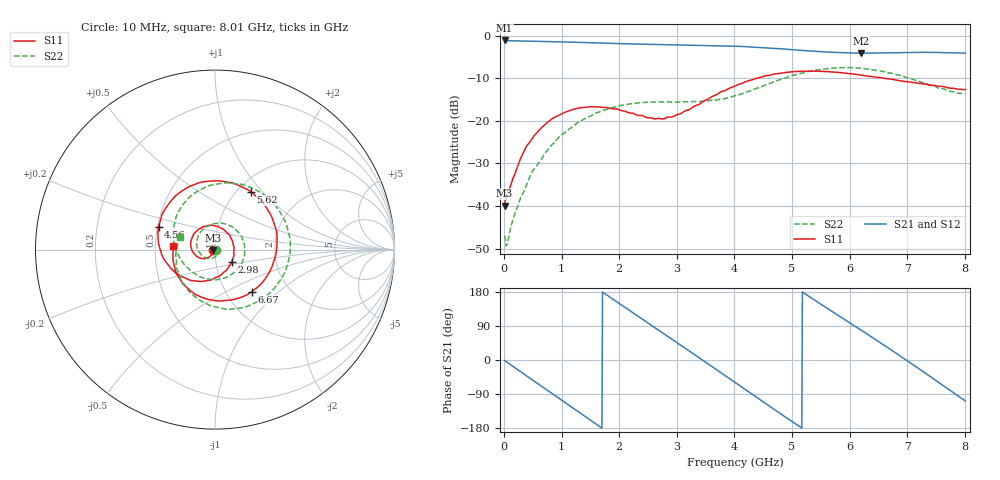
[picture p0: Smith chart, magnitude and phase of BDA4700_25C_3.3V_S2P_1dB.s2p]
!Agilent Technologies,E5071B,MY42404982,A.09.10
!Date: Mon Oct 20 18:03:23 2025
!Data & Calibration Information:
!Freq	S11:SOLT2(ON)	S21:SOLT2(ON)	S12:SOLT2(ON)	S22:SOLT2(ON)
# Hz S RI R 50
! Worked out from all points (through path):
!   801 points, 10 MHz to 8.01 GHz, reference 50 ohm
!   highest |S21| = -1.12 dB at 10 MHz (marker M1); lowest = -4.1 dB at 6.2 GHz (marker M2)
!   group delay of S21, straight-line fit = 286 ps
!   lowest |S11| = -39.9 dB at 10 MHz (marker M3), VSWR 1.02, Z = 49 - j0.224 ohm
!   |S11| at or under -10 dB: start of sweep to 4.387 GHz; 6.606 GHz to end of sweep
!   |S22| runs from -49.4 to -7.5 dB; largest |S21 - S12| = 0.01
!   S11 on the Smith chart (normalised r, x): 10 MHz: 0.98, -0.00; 2.98 GHz: 1.19, -0.17; 4.56 GHz: 0.51, +0.15; 5.62 GHz: 1.15, +0.87; 6.67 GHz: 1.32, -0.68; 8.01 GHz: 0.62, +0.03
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1e7  -0.00986 -0.00229  0.8784 -0.0191  0.8781 -0.0194  0.00438 -0.000888
3.6e8  -0.0267 -0.0371  0.6748 -0.5401  0.6742 -0.54  0.0134 -0.00817
7.1e8  -0.0759 -0.0489  0.2108 -0.8274  0.2111 -0.8278  -0.00118 -0.0411
1.02e9  -0.1217 -0.0153  -0.2657 -0.801  -0.2658 -0.8012  -0.0531 -0.0454
1.35e9  -0.1323 0.0537  -0.6653 -0.4997  -0.6655 -0.4999  -0.0999 0.0153
1.63e9  -0.0962 0.1095  -0.8141 -0.1091  -0.8141 -0.1093  -0.0842 0.0933
1.92e9  -0.0293 0.135  -0.7481 0.3114  -0.7485 0.3109  -0.00287 0.1452
2.32e9  0.0644 0.0962  -0.3508 0.7148  -0.3507 0.7149  0.129 0.0979
2.68e9  0.1058 0.0134  0.15 0.7729  0.1487 0.7725  0.1636 -0.0339
2.98e9  0.0922 -0.0709  0.5209 0.5802  0.5199 0.5795  0.1058 -0.1283
3.48e9  -0.0261 -0.1698  0.7668 -0.0506  0.767 -0.0507  -0.0585 -0.1603
4.01e9  -0.2254 -0.124  0.3849 -0.6455  0.3857 -0.6446  -0.1867 -0.0626
4.56e9  -0.3139 0.1264  -0.3244 -0.6412  -0.3238 -0.6422  -0.227 0.1382
4.97e9  -0.1877 0.3242  -0.6426 -0.2441  -0.643 -0.2465  -0.1139 0.3145
5.35e9  0.0377 0.3814  -0.628 0.2014  -0.6293 0.1977  0.1132 0.3676
5.62e9  0.1994 0.3223  -0.4583 0.4499  -0.4583 0.4499  0.2815 0.2985
6.2e9  0.3434 0.00255  0.1208 0.6101  0.1292 0.6114  0.4067 -0.0742
6.67e9  0.206 -0.2337  0.5346 0.3318  0.5353 0.3299  0.2053 -0.3048
6.68e9  0.2012 -0.2374  0.5399 0.3214  0.5417 0.3207  0.1995 -0.3072
7.25e9  -0.0952 -0.2562  0.5629 -0.2998  0.5627 -0.2997  -0.1146 -0.2593
7.63e9  -0.217 -0.1293  0.2364 -0.5855  0.2358 -0.5867  -0.2161 -0.0996
8.01e9  -0.2313 0.0219  -0.1957 -0.5914  -0.1936 -0.5923  -0.1954 0.0723
